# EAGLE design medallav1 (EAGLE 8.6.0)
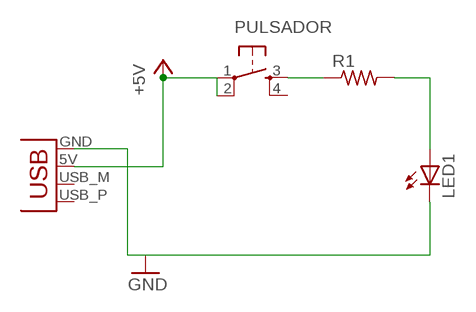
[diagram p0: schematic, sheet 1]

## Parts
LED1  LED5MM  [LED5MM]
PULSADOR  TAC_SWITCHPTH  [TACTILE-PTH]
R1  R-US_0207/10  [0207/10]
X1  USBPCB  [USB-A-PCB]

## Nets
+5V: PULSADOR.1 PULSADOR.2 X1.5V(VBUS)
GND: LED1.K(C) X1.GND
N$1: LED1.A R1.2
N$2: PULSADOR.3 R1.1
Unconnected: PULSADOR.4 X1.USB_M(D-) X1.USB_P(D+)

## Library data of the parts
LED1 = led:LED: LED
PULSADOR = SparkFun-Retired:TAC_SWITCH: Momentary Switch Button commonly used for reset or general input. Spark Fun Electronics SKU : COM-00097 SMT- SWCH-08247
R1 = resistor:R-US_: RESISTOR, American symbol
X1 = SparkFun:USB: USB Connectors USB-B-PTH is fully proven SKU : PRT-00139 USB-miniB is fully proven SKU : PRT-00587 USB-A-PCB is untested. USB-A-H is throughly reviewed, but untested. Spark Fun Electronics SKU : PRT-00437 USB-B-SMT is throughly reviewed, but untested. Needs silkscreen touching up. USB-A-S has not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

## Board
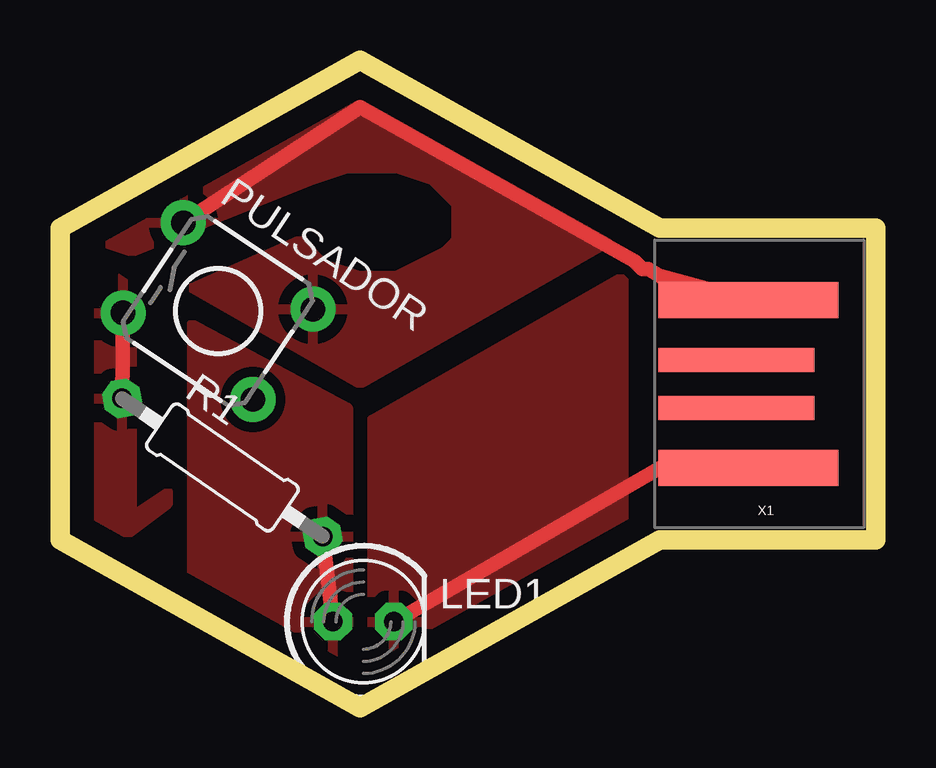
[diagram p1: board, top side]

Size 34 x 27 mm. Coordinates in mm from the lower left corner, seen from the top.
Outline: 34,20 25,20 12.5,27 0,20 0,7 12.5,0 25,7 34,7 34,20
Copper layers (1*16): Top 0.035mm / dielectric 1.5mm / Bottom 0.035mm
Design rules "Fablab U. de Chile": minimum track width 0.6mm, minimum drill 0.6mm, track to track 0.3mm, track to pad 0.3mm, pad to pad 0.3mm, via to via 0.3mm, smd to smd 0.3mm, copper to edge 1mm, drill to drill 0.3mm, minimum pad ring 15mil, minimum via ring 10mil, stop-mask expansion 10mil, vias tented up to drill 0mil, thermal gap 20mil

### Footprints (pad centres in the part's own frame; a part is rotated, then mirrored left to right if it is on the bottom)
LED5MM = drill 0.813 octagon: A -1.27,0; K 1.27,0
TACTILE-PTH = drill 1.016 pad 1.88: 1 -3.251,2.261; 2 3.251,2.261; 3 -3.251,-2.261; 4 3.251,-2.261
0207/10 = drill 0.813 octagon: 1 -5.08,0; 2 5.08,0
USB-A-PCB = smd 7.5 x 1.5: 5V -0.2,-3.5; GND -0.2,3.5 | smd 6.5 x 1: USB_M 0.3,-1; USB_P 0.3,1

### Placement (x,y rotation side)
LED1  12.65,3.58 0 top
PULSADOR  6.59,16.53 326.3 top
R1  6.77,10.01 325.4 top
X1  28.5,13.5 180 top

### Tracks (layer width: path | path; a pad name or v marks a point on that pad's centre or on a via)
+5V
  Top 0.61: X1.5V 25,18 24.54,18.29 24.29,18.29 23.96,18.62 20.91,20.33 | 20.91,20.33 | 20.91,20.33 12.5,25.04 PULSADOR.1
  pour Top (isolate 0.406): 23,19.5 12.5,25.5 1.5,19.5 3,19 10.5,22 12,22.5 14,22.5 15.5,22 16.5,21 16.5,19.5 16,19 14,18 12.5,18 11,18.5 10,19.5 5.5,17.5 12.5,13.5
GND
  Top 0.61: LED1.K 25,10 X1.GND
  pour Top (isolate 0.406): 23.5,18 13,12 13,1.5 23.5,7.5
N$1
  Top 0.61: R1.2 LED1.A
  pour Top (isolate 0.406): 12,1.5 5.5,5 5.5,16 12,12.5
N$2
  Top 0.61: R1.1 PULSADOR.3
  pour Top (isolate 0.406): 1.5,18.5 1.5,7.5 2.5,7 4.5,8.5 4.5,9 3,8 3,17.5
